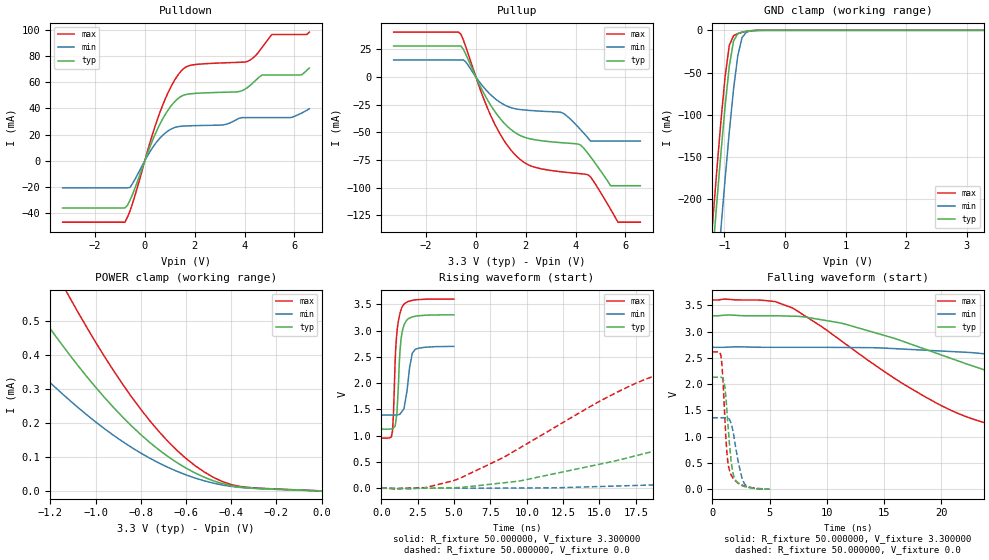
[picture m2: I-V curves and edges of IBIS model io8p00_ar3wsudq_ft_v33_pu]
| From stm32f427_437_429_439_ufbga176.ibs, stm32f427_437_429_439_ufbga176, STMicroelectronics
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|   Model io8p00_ar3wsudq_ft_v33_pu
[Model]  io8p00_ar3wsudq_ft_v33_pu
Model_type I/O
Polarity   Non-Inverting
Enable   Active-Low
Vinl =   0.990000V
Vinh =   2.310000V
Vmeas =  1.650000V
Cref =   50.000000pF
Rref =   100.000000M
Vref =   0.0V
C_comp   3.857500pF   3.762100pF   3.941700pF
[Temperature Range]   25.000000   0.125000k   -40.000000
[Pullup Reference]   3.300000V   2.700000V   3.600000V
[Pulldown Reference]   0.0V   0.0V   0.0V
[POWER Clamp Reference]   3.300000V   2.700000V   3.600000V
[GND Clamp Reference]   0.0V   0.0V   0.0V
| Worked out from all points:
|   slope of the pulldown table from 0 to 0.495 V, typ, clamps not added: 20.9 ohm
|   slope of the pullup table from 0 to 0.495 V, typ, clamps not added: 22.6 ohm
|   GND clamp passes 1 mA (typ) near -0.62 V on its own axis
|   POWER clamp passes 1 mA (typ) near -1.88 V on its own axis
|   rising waveform, R_fixture 50.000000, V_fixture 3.300000: 20-80 % time 275ps typ, 397ps min, 272ps max; typ from 1.12 V to 3.3 V
|   rising waveform, R_fixture 50.000000, V_fixture 0.0: 20-80 % time 19.7ns typ, 51.8ns min, 10.4ns max; typ from 0.001 V to 2.13 V
|   falling waveform, R_fixture 50.000000, V_fixture 3.300000: 20-80 % time 18.7ns typ, 38.7ns min, 11.3ns max; typ from 3.3 V to 1.12 V
|   falling waveform, R_fixture 50.000000, V_fixture 0.0: 20-80 % time 512ps typ, 708ps min, 436ps max; typ from 2.13 V to 0.001 V
[Pulldown]
|Voltage   I(typ)   I(min)   I(max)
-3.3V     -36.18mA   -20.77mA   -47.07mA
-800mV    -36.18mA   -20.77mA   -47.07mA
-600mV    -30.5mA    -20.52mA   -38.69mA
700mV     31.4mA     19.11mA    41.71mA
1.2V      45.15mA    25.37mA    61.75mA
1.6V      50.35mA    26.5mA     71.06mA
3.1V      52.28mA    27.26mA    74.76mA
4.1V      55.65mA    32.9mA     75.79mA
4.7V      65.5mA     32.9mA     86.49mA
5.1V      65.5mA     32.9mA     96.53mA
6.3V      65.8mA     36.47mA    96.53mA
6.6V      70.85mA    39.68mA    98.34mA
[Pullup]
|Voltage   I(typ)   I(min)   I(max)
-3.3V     28mA       15.42mA    40.61mA
-700mV    28mA       15.42mA    40.61mA
-400mV    20.3mA     13.47mA    26.92mA
600mV     -25.77mA   -16.23mA   -35.13mA
1.6V      -50.64mA   -28.8mA    -70.96mA
2.3V      -56.49mA   -30.48mA   -81.16mA
3.5V      -59.52mA   -32.72mA   -85.91mA
4.2V      -61.52mA   -47.6mA    -87.45mA
4.5V      -69.2mA    -55.14mA   -88.43mA
5.4V      -98.3mA    -57.9mA    -119.4mA
5.7V      -98.3mA    -57.9mA    -131.3mA
6.6V      -98.3mA    -57.9mA    -131.3mA
[GND_clamp]
|Voltage   I(typ)   I(min)   I(max)
-3.3V     -2.333A    -2.407A    -2.313A
-1.2V     -270.2mA   -361.4mA   -232.1mA
-1.13V    -207.3mA   -298.1mA   -169mA
-1.06V    -146.7mA   -236.2mA   -108.8mA
-990mV    -90.18mA   -176.4mA   -54.96mA
-920mV    -42.21mA   -120mA     -17.68mA
-850mV    -12.57mA   -69.47mA   -6.265mA
-780mV    -3.971mA   -30.01mA   -3.886mA
-710mV    -2.1mA     -8.615mA   -2.382mA
-640mV    -1.148mA   -2.283mA   -1.22mA
-570mV    -524uA     -821.5uA   -476.8uA
3.28V     0A         0A         0A
[POWER_clamp]
|Voltage   I(typ)   I(min)   I(max)
-3.28V    1.18mA     571.5uA    1.791mA
-3.08V    1.154mA    558.1uA    1.753mA
-1.84V    973.4uA    557.7uA    1.433mA
-1.32V    593.1uA    370.2uA    831.6uA
-1.28V    553.9uA    355.9uA    778.7uA
-1.12V    406uA      270.4uA    577.3uA
-960mV    275.2uA    183.2uA    395.9uA
-800mV    166.2uA    111.7uA    240.7uA
-680mV    101.4uA    69.6uA     146.3uA
-560mV    53.02uA    38.04uA    74.62uA
-360mV    11.49uA    10.29uA    13.1uA
0V        0A         0A         0A
[Ramp]
| variable   typ   min   max
dV/dt_r  1.27717/19.67360n   0.81585/51.90639n   1.56688/10.37938n
dV/dt_f  1.30638/18.66053n   0.78432/38.81400n   1.58716/11.31251n
R_load = 50.000000
[Rising Waveform]
R_fixture= 50.000000
V_fixture= 3.300000
V_fixture_min= 2.700000
V_fixture_max= 3.600000
|time   V(typ)   V(min)   V(max)
0s        1.125V     1.393V     954.7mV
760.8ps   1.133V     1.393V     1.078V
840.8ps   1.152V     1.393V     1.459V
1.041ns   1.366V     1.397V     2.872V
1.281ns   2.6V       1.411V     3.323V
1.441ns   2.984V     1.471V     3.456V
1.562ns   3.102V     1.522V     3.502V
2.132ns   3.259V     2.571V     3.575V
2.332ns   3.272V     2.645V     3.586V
4.985ns   3.3V       2.7V       3.6V
[Rising Waveform]
R_fixture= 50.000000
V_fixture= 0.0
V_fixture_min= 0.0
V_fixture_max= 0.0
|time   V(typ)   V(min)   V(max)
0s        1.089mV    1.043mV    1.137mV
3.003ns   3.586mV    2.206mV    13.48mV
5.506ns   16.5mV     2.824mV    204.9mV
19.52ns   761.2mV    70.55mV    2.204V
26.03ns   1.204V     158.5mV    2.467V
34.53ns   1.721V     298.3mV    2.56V
55.06ns   2.058V     673.9mV    2.607V
86.59ns   2.117V     1.11V      2.613V
117.1ns   2.129V     1.3V       2.613V
249.2ns   2.13V      1.36V      2.613V
[Falling Waveform]
R_fixture= 50.000000
V_fixture= 3.300000
V_fixture_min= 2.700000
V_fixture_max= 3.600000
|time   V(typ)   V(min)   V(max)
0s        3.3V       2.7V       3.6V
7.007ns   3.292V     2.7V       3.447V
16.52ns   2.823V     2.668V     2.024V
22.52ns   2.36V      2.601V     1.352V
32.03ns   1.709V     2.411V     1.068V
39.04ns   1.4V       2.25V      1.023V
46.55ns   1.274V     2.069V     998.2mV
65.07ns   1.18V      1.698V     968.6mV
86.59ns   1.146V     1.526V     957.1mV
249.2ns   1.125V     1.393V     954.7mV
[Falling Waveform]
R_fixture= 50.000000
V_fixture= 0.0
V_fixture_min= 0.0
V_fixture_max= 0.0
|time   V(typ)   V(min)   V(max)
0s        2.13V      1.36V      2.613V
780.8ps   2.127V     1.359V     2.49V
860.9ps   2.12V      1.359V     2.294V
1.091ns   1.943V     1.359V     1.358V
1.261ns   1.523V     1.355V     721.2mV
1.411ns   1.092V     1.343V     438mV
1.622ns   574.7mV    1.264V     282.6mV
1.962ns   199.3mV    894.2mV    170.1mV
2.773ns   53.27mV    116.8mV    62.1mV
4.985ns   1.089mV    1.043mV    1.137mV
